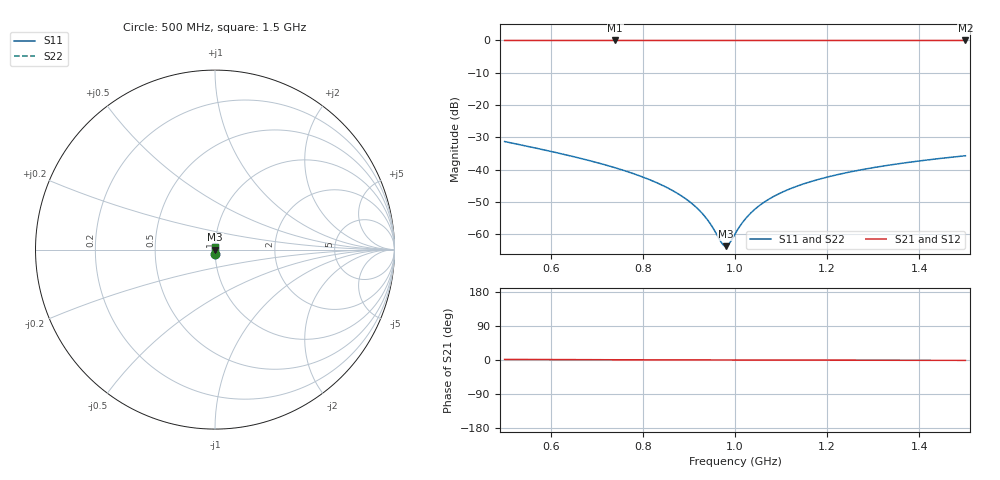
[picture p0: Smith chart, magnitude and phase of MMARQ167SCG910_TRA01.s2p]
! MMARQ167SCG910_TRA01  S-PARAMETER MODEL  ( General Type )
! Model Generated by TAIYO YUDEN Corporation (http://www.ty-top.com)
! Version 1.0
! TAIYO YUDEN Control No. 150609
! Copyright(c) 2015 TAIYO YUDEN CO.,LTD. All Rights Reserved.
! Product Description (link to TY-COMPAS)
! https://ds.yuden.co.jp/TYCOMPAS/or/detail?pn=MMARQ167SCG910JTRA01&u=M
! Products Name : Multilayer Ceramic Capacitors
! Characteristics :
!  Capacitance : 91 pF , Rated Voltage : 250V , TCC : CG / C0G
!  Case Size : 1.6 x 0.8 / 0.063 x 0.031 [mm/inch] , Thickness : 0.7 / 0.028 [mm/inch]
!  (Conditions: Temperature = 25 degC , DC Bias Current/Voltage = 0A / 0V)
! External Node Assignments :
!  1  o---| |---o  2
! GND o---------o GND
! Frequency Range : 500MHz  -  1.5GHz  [ 401 STEP ]
# MHz S RI R 50
! Freq[MHz].  S11 Real  S11 Imag  S21 Real  S21 Imag  S12 Real  S12 Imag  S22 Real  S22 Imag
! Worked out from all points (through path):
!   401 points, 500 MHz to 1.5 GHz, reference 50 ohm
!   highest |S21| = 0.00 dB at 740 MHz (marker M1); lowest = 0.0 dB at 1.5 GHz (marker M2)
!   lowest |S11| = -63.7 dB at 980 MHz (marker M3), VSWR 1.00, Z = 50.1 - j2.52e-05 ohm
!   |S11| at or under -10 dB: start of sweep to end of sweep
!   |S22| runs from -63.7 to -31.3 dB; largest |S21 - S12| = 0
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500  0.00114 -0.0272  0.9989 0.0272  0.9989 0.0272  0.00114 -0.0272
667.5  0.000688 -0.0148  0.9993 0.0148  0.9993 0.0148  0.000688 -0.0148
740  0.000623 -0.0107  0.9994 0.0107  0.9994 0.0107  0.000623 -0.0107
792.5  0.000603 -0.00802  0.9994 0.00802  0.9994 0.00802  0.000603 -0.00802
835  0.0006 -0.00603  0.9994 0.00603  0.9994 0.00603  0.0006 -0.00603
880  0.000608 -0.00404  0.9994 0.00404  0.9994 0.00404  0.000608 -0.00404
915  0.000619 -0.00257  0.9994 0.00257  0.9994 0.00257  0.000619 -0.00257
930  0.000626 -0.00196  0.9994 0.00196  0.9994 0.00196  0.000626 -0.00196
942.5  0.000632 -0.00146  0.9994 0.00146  0.9994 0.00146  0.000632 -0.00146
972.5  0.000649 -0.000288  0.9994 0.000288  0.9994 0.000288  0.000649 -0.000288
980  0.000654 -2.52e-07  0.9993 2.52e-07  0.9993 2.52e-07  0.000654 -2.52e-07
987.5  0.000659 0.000285  0.9993 -0.000285  0.9993 -0.000285  0.000659 0.000285
1000  0.000667 0.000756  0.9993 -0.000756  0.9993 -0.000756  0.000667 0.000756
1012.5  0.000676 0.00122  0.9993 -0.00122  0.9993 -0.00122  0.000676 0.00122
1027.5  0.000687 0.00177  0.9993 -0.00177  0.9993 -0.00177  0.000687 0.00177
1045  0.000702 0.0024  0.9993 -0.0024  0.9993 -0.0024  0.000702 0.0024
1062.5  0.000716 0.00303  0.9993 -0.00303  0.9993 -0.00303  0.000716 0.00303
1107.5  0.000758 0.00458  0.9992 -0.00458  0.9992 -0.00458  0.000758 0.00458
1167.5  0.000821 0.00658  0.9992 -0.00658  0.9992 -0.00658  0.000821 0.00658
1242.5  0.000911 0.00895  0.9991 -0.00895  0.9991 -0.00895  0.000911 0.00895
1335  0.00104 0.0117  0.999 -0.0117  0.999 -0.0117  0.00104 0.0117
1500  0.00129 0.0163  0.9987 -0.0163  0.9987 -0.0163  0.00129 0.0163
